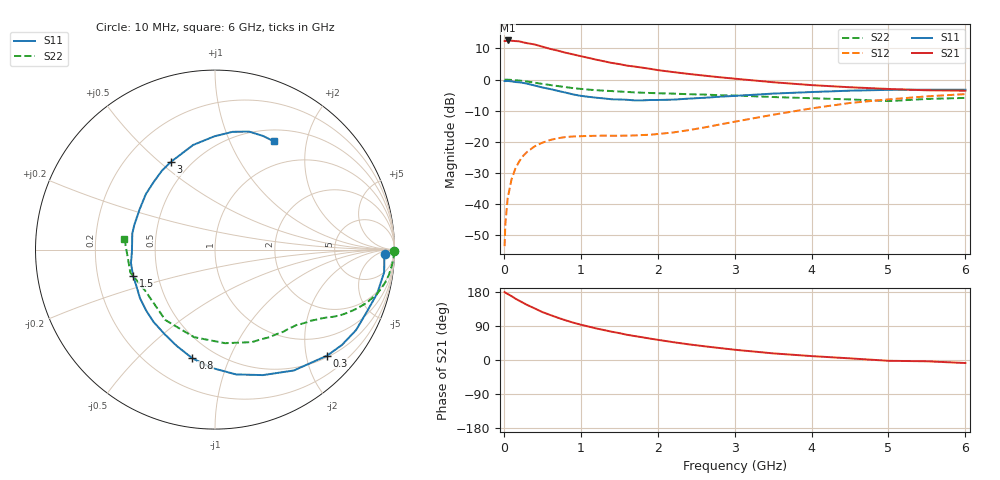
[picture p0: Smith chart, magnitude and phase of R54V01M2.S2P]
! SIEMENS Small Signal Semiconductors
! BFR183
! Si NPN RF Bipolar Junction Transistor in SOT23
! VCE = 4 V  IC = 1.2 mA
! Common Emitter S-Parameters:  May  1996
# GHz  S  MA  R  50
!  f  S11  S21  S12  S22
! GHz  MAG  ANG  MAG  ANG  MAG  ANG  MAG  ANG
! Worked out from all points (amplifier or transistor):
!   36 points, 10 MHz to 6 GHz, reference 50 ohm
!   highest |S21| = 12.6 dB at 50 MHz (marker M1)
!   |S21| within 3 dB of that: start of sweep to 653.8 MHz
!   unconditionally stable (mu >= 1): 1.607 GHz to 2.904 GHz
!   at 250 MHz: K = 0.17, MSG = 18.3 dB, |S12| = -24.6 dB
!   at 1.4 GHz: K = 0.89, MSG = 11.7 dB, |S12| = -18.1 dB
!   at 6 GHz: K = 0.94, MSG = 0.5 dB, |S12| = -4.7 dB
!   S11 on the Smith chart (normalised r, x): 10 MHz: 30, -15; 300 MHz: 0.53, -2.41; 800 MHz: 0.38, -0.74; 1.5 GHz: 0.36, -0.14; 3 GHz: 0.39, +0.54; 6 GHz: 0.65, +1.48
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0.01  0.9475 -1.5  4.176 179.2  0.0021 90.1  0.9979 -0.5
0.02  0.9447 -2.9  4.154 177.6  0.0048 85.3  0.9963 -1.1
0.05  0.9508 -7.6  4.257 174.2  0.0124 85.0  0.9958 -2.8
0.1  0.9362 -15.1  4.213 168.6  0.0249 81.1  0.9878 -5.5
0.15  0.9137 -22.5  4.161 162.0  0.0372 76.2  0.9791 -8.3
0.2  0.9048 -29.7  4.118 156.4  0.0484 72.4  0.9663 -10.9
0.3  0.8597 -43.4  3.855 145.6  0.0684 65.0  0.9339 -15.5
0.4  0.804 -56.9  3.673 136.2  0.0845 58.1  0.8927 -19.6
0.5  0.7485 -69.1  3.383 126.6  0.0967 52.2  0.8516 -22.9
0.7  0.66 -91.3  2.922 111.7  0.114 43.6  0.7877 -27.7
0.8  0.6189 -101.7  2.709 104.9  0.1192 40.2  0.7576 -29.6
0.9  0.5777 -111.6  2.542 98.7  0.1218 38.0  0.7297 -31.2
1.1  0.5287 -130.4  2.235 88.3  0.1244 35.0  0.6905 -34.3
1.3  0.498 -147.1  1.972 79.1  0.1258 33.8  0.664 -36.7
1.5  0.4793 -162.4  1.775 71.0  0.125 34.8  0.6433 -39.5
1.8  0.4634 175.2  1.555 60.0  0.1284 39.6  0.6159 -43.4
2.2  0.4761 151.9  1.322 47.1  0.1412 47.6  0.5953 -50.2
3  0.5466 116.9  1.035 27.1  0.2103 56.5  0.5549 -68.3
3.5  0.5956 101.8  0.907 17.5  0.2723 54.7  0.5244 -83.9
4.5  0.6635 81.5  0.753 4.3  0.4209 42.3  0.4801 -125.2
5.5  0.6876 67.0  0.673 -3.4  0.5377 25.8  0.4885 -164.9
6  0.6867 61.4  0.663 -8.0  0.5845 15.9  0.5077 173.3
